FUNCTION_BLOCK FB42
TITLE =Get All Digital Outputs
//*****************************************************************************
//* maxon motor ag
//* R&D
//* all rights reserved
//*****************************************************************************
//* Summary:  Read all digital outputs
//*
//* Remarks:
//*
//* Created under: STEP7 REV5.2+SP1
//*****************************************************************************
//* History:
//* 19.05.2004 | INA   first release
//*
//*
//*****************************************************************************
//

AUTHOR:INA
FAMILY:I_O_Mode
NAME:GetDigOu
VERSION:00.01


VAR_INPUT

Read : BOOL //A rising edge start the command

  NodeID : BYTE //Adress of the maxon device

END_VAR
VAR_OUTPUT
  Done : BOOL //Data valid flag is TRUE if data were available

  Err : BOOL //Error flag is TRUE if an Error has occured, see ErrNo for more details

  ErrNo : DINT //Contains detailed error information

  Outputs : WORD //State of all digital outputs

END_VAR
VAR
  xEdgeMerker : BOOL //Edge Merker

  xEdgeFlag : BOOL //Edge Flag

  xStep : INT
END_VAR

BEGIN

NETWORK
TITLE = Activate the service function
//

// SDO Read "Get All Digital Outputs"

       U    #Read
       FP   #xEdgeFlag                   // recognize a positiv edge of the Read signal
       =    #xEdgeMerker                 // and set the xEdgeMerker for one cycle to true

       L    #xStep
       L    0
       ==I
       U    #xEdgeMerker
       SPB  nstp                         // iStep = 1 -> fnc1

       L    #xStep                       // jump list
       SPL  List
       SPA  rdef
       SPA  fnc1
       SPA  fncE
List  :SPA  rdef

rdef  :NOP  0
       R    #Done                        // reset Done
       R    #Err                         // reset Error
       L    0
       T    #xStep                       // iStep = 0
       SPA  end

fnc1  :NOP  0
       CALL FC1
         NodeID:=#NodeID
         Index:=DW#16#00002078
         SubIndex:=DW#16#00000001
         RET_VAL:=#Done
         Err:=#Err
         ErrNo:=#ErrNo

       L    DB219.DBW10
       T    #Outputs

fncE  :NOP  0
       L    0
       T    #xStep
       SPA  end

nstp  :NOP  0
       L    #xStep
       INC            1
       T    #xStep

end   :NOP  0
END_FUNCTION_BLOCK
